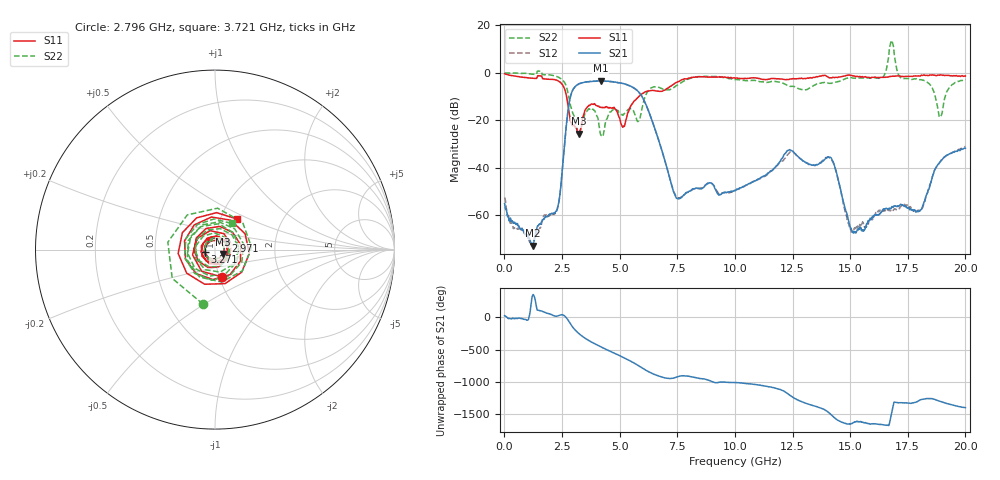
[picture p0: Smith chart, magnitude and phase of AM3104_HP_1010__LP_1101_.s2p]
!Created with skrf (http://scikit-rf.org).
# Hz S RI R 50.0
!freq ReS11 ImS11 ReS21 ImS21 ReS12 ImS12 ReS22 ImS22
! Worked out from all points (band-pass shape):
!   1601 points, 10 MHz to 20 GHz, reference 50 ohm
!   highest |S21| = -3.36 dB at 4.183 GHz (marker M1); lowest = -72.8 dB at 1.222 GHz (marker M2)
!   |S21| within 3 dB of the highest: 3.025 GHz to 5.617 GHz (2.592 GHz wide, 60 % of centre)
!   lowest |S11| = -25.7 dB at 3.221 GHz (marker M3), VSWR 1.11, Z = 54.8 - j2.65 ohm
!   |S11| at or under -10 dB: 2.698 GHz to 5.827 GHz (3.129 GHz wide, 73.4 % of centre)
!   |S22| runs from -26.8 to 13.6 dB; largest |S21 - S12| = 0.07
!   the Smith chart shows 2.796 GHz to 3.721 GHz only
!   S11 on the Smith chart (normalised r, x): 2.796 GHz: 1.03, -0.32; 2.971 GHz: 1.12, +0.11; 3.271 GHz: 0.89, -0.02; 3.721 GHz: 1.19, +0.43
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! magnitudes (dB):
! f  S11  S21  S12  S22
! 10 MHz  -0.4  -55.1  -52.5  -0.1
! 1.222 GHz  -2.3  -72.8  -73.0  -0.6
! 2.296 GHz  -3.2  -57.4  -57.4  -1.7
! 2.796 GHz  -16.1  -13.5  -13.6  -10.2
! 2.971 GHz  -22.3  -7.1  -7.1  -17.1
! 3.221 GHz  -25.7  -4.7  -4.8  -25.9
! 3.271 GHz  -24.5  -4.5  -4.6  -24.7
! 3.346 GHz  -22.5  -4.2  -4.3  -22.7
! 3.721 GHz  -13.6  -3.6  -3.7  -15.3
! 4.183 GHz  -14.6  -3.4  -3.4  -26.2
! 5.145 GHz  -22.8  -4.5  -4.5  -17.9
! 5.795 GHz  -10.4  -7.7  -7.8  -20.5
! 6.682 GHz  -7.7  -28.0  -28.1  -6.0
! 7.506 GHz  -3.9  -52.9  -52.6  -5.2
! 10.01 GHz  -2.3  -49.7  -49.5  -2.9
! 13.34 GHz  -2.2  -38.9  -38.9  -5.9
! 14.2 GHz  -2.1  -36.4  -36.6  -4.4
! 15.15 GHz  -1.3  -66.7  -66.2  -2.2
! 16.68 GHz  -1.6  -57.4  -57.9  7.3
! 18.03 GHz  -1.4  -58.2  -57.8  -2.9
! 18.91 GHz  -0.8  -37.3  -37.4  -18.5
! 20 GHz  -1.3  -31.7  -31.1  -2.8
